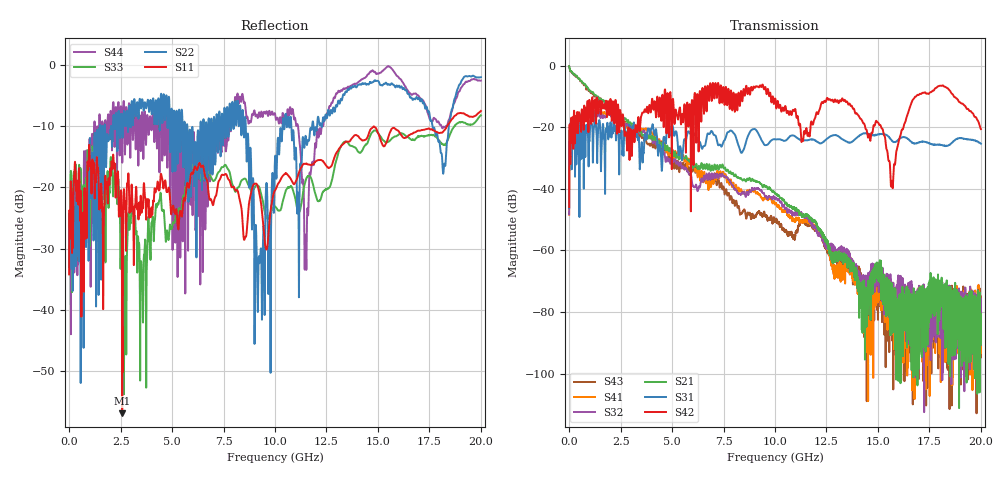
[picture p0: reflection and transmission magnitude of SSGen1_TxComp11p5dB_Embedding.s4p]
! Save cascaded4-port  S-parameter
# GHz S RI R 50
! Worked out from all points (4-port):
!   6401 points, 300 kHz to 20 GHz, reference 50 ohm
!   strongest paths, dB at 300 kHz, 5 GHz, 10 GHz, 15 GHz, 20 GHz:
!     S42: -45.9, -20.7, -10.7, -18.5, -20.6
!     S31: -46.2, -19.2, -23.9, -22.3, -25.3
!     S21: -0.2, -27.5, -41.5, -67.8, -84.6
!     S32: -48.3, -30.1, -43.1, -65.8, -84.3
!     S41: -48.4, -27.7, -45.1, -70.5, -88.4
!     S43: -0.2, -31.0, -50.7, -82.5, -76.3
!   lowest |S11| = -56.9 dB at 2.578 GHz (marker M1), VSWR 1.00, Z = 50.1 + j0.0792 ohm
!   |S11| at or under -10 dB: start of sweep to 18.36 GHz
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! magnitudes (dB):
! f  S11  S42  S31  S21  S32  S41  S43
! 300 kHz  -34.2  -45.9  -46.2  -0.2  -48.3  -48.4  -0.2
! 2.578 GHz  -56.9  -17.5  -27.4  -16.5  -18.5  -17.7  -17.5
! 8.241 GHz  -21.3  -9.0  -26.1  -36.4  -41.8  -39.7  -45.8
! 9.206 GHz  -20.4  -7.0  -22.2  -37.8  -40.0  -41.8  -47.6
! 11.52 GHz  -16.1  -20.4  -24.3  -48.5  -49.2  -49.9  -51.4
! 15.68 GHz  -10.4  -37.6  -24.4  -71.8  -74.2  -77.8  -79.1
! 20 GHz  -7.5  -20.6  -25.3  -84.6  -84.3  -88.4  -76.3
